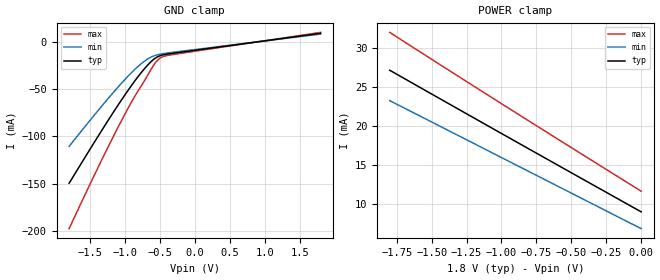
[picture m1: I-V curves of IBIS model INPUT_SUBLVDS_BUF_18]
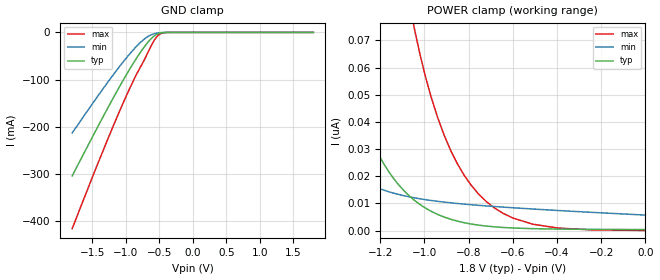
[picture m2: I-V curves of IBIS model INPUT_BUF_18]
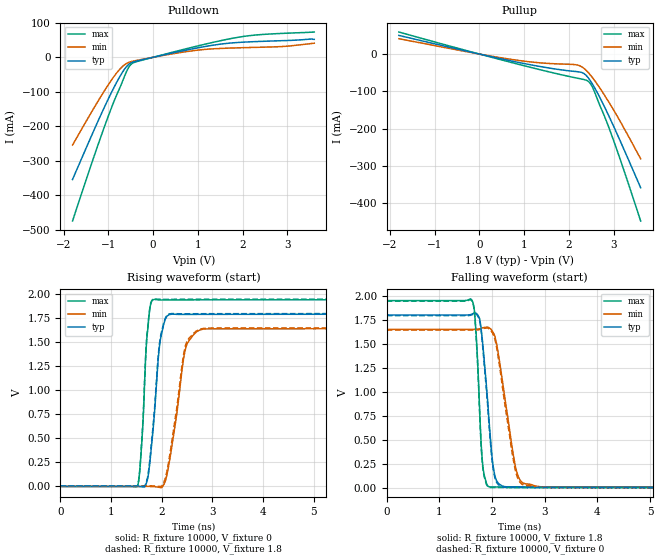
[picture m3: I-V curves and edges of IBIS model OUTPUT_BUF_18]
| TEXAS INSTRUMENTS INCORPORATED
| DLP Products
| IBIS Model of D4885XT7SV
| DLP2010 DMD
| This device can be powered at the following Vccs:
|  1.8 volt Vcc
| This file provides unique models under the [Model Selector] for each Vcc.
| For operation at a specific Vcc, select the appropriate model after each
| [Model Selector] keyword.
[IBIS Ver]   3.2
[Comment char]  |_char
[File Name]   dlp2010dmd_ibis.ibs
[File Rev]   1.0 | f_die
[Date]   December 3, 2012
[Source]   Data created from TI-SPICE simulations at TI-DLP.
[Notes]   The following is an IBIS list for the P2_WVGA.
##notes##|
[Disclaimer] Property of Texas Instruments Incorporated.  Unauthorized
   reproduction and/or distribution is strictly prohibited.
   This product is protected under copyright law.
   Created  2012, (C) Copyright  2012, Texas Instruments
   Incorporated, All Rights Reserved
   UNLESS THERE IS A SIGNED, WRITTEN AGREEMENT TO THE
   CONTRARY, TEXAS INSTRUMENTS (TI) IS PROVIDING THE IBIS
   MODELS  AND WITHOUT ANY WARRANTY, EXPRESSED OR
   IMPLIED.  TI assumes no liability for:
   1) the accuracy of the IBIS models provided to your
   company;
   2) the proper functioning of these IBIS Models in your
   design or for any resulting applications; or
   3) infringement of patents, copyrights or intellectual
   property rights resulting from your use of these IBIS
   models.
   TI provides IBIS Models as a service to our customers.
   You and your company shall not distribute, sell or give
   these models to anyone else without prior written
   permission from TI.
   TI reserves the right to make changes to our products or
   to discontinue any semiconductor product or service
   without notice, and advises our customers to obtain the
   latest version of relevant information to verify, before
   placing orders, that the information being relied on is
   current.
   Please be aware that your receipt and use of the IBIS
   information provided shall serve as acceptance of these
   terms and conditions.  If you do not accept these terms,
   you should return or destroy the IBIS models and any
   other accompanying information immediately.
| Component DLP2010 40-pin PGA
[Component]   DLP2010
[Manufacturer]   Texas Instruments, Inc.
[Package]
|   typ   min   max
R_pkg   1.276e+00   6.417e-01   1.439e+00
L_pkg   5.442e-09   3.319e-09   6.457e-09
C_pkg   2.002e-12   1.417e-12   2.333e-12
[Pin]   signal_name   model_name   R_pin   L_pin   C_pin
G1   VDDI   POWER
G2   VDDI   POWER
G3   D_P<0>   INPUT_SUB_LVDS_BUF   1.398e+00   5.548e-09   2.270e-12
G4   D_N<0>   INPUT_SUB_LVDS_BUF   1.425e+00   5.892e-09   2.333e-12
G5   VDDI   POWER
G6   VDDI   POWER
G7   D_P<1>   INPUT_SUB_LVDS_BUF   1.427e+00   6.052e-09   1.970e-12
G8   D_N<1>   INPUT_SUB_LVDS_BUF   1.439e+00   6.208e-09   1.878e-12
G9   VSS   GND
G10   VSS   GND
G11   LS_RDATA   OUTPUT_BUF   1.414e+00   6.457e-09   2.308e-12
G12   DMD_DEN_ARSTZ INPUT_BUF   9.967e-01   4.805e-09   1.900e-12
G13   VSS   GND
G14   VSS   GND
G15   VSS   GND
G16   VSS   GND
G17   VSS   GND
G18   LS_WDATA   INPUT_BUF   6.417e-01   3.319e-09   1.454e-12
G19   LS_CLK   INPUT_BUF   6.511e-01   3.395e-09   1.417e-12
G20   VDD   POWER
H1   D_N<3>   INPUT_SUB_LVDS_BUF   1.386e+00   5.227e-09   2.120e-12
H2   D_P<3>   INPUT_SUB_LVDS_BUF   1.404e+00   5.656e-09   1.942e-12
H3   VSS   GND
H4   VSS   GND
H5   D_N<2>   INPUT_SUB_LVDS_BUF   1.422e+00   5.823e-09   2.144e-12
H6   D_P<2>   INPUT_SUB_LVDS_BUF   1.413e+00   5.770e-09   2.030e-12
H7   VSS   GND
H8   VSS   GND
H9   DCLK_N   INPUT_SUB_LVDS_BUF   1.425e+00   5.952e-09   2.136e-12
H10   DCLK_P   INPUT_SUB_LVDS_BUF   1.428e+00   6.083e-09   2.128e-12
H11   VSS   GND
H12   VSS   GND
H13   VOFFSET   POWER
H14   VDD   POWER
H15   VDD   POWER
H16   VDD   POWER
H17   VBIAS   POWER
H18   VRESET   POWER
H19   VDD   POWER
H20   VDD   POWER
| NOTE:  The [Diff Pin] section is commented out because the ibischk3 program
|   currently flags it as an Error when it shouldn't
| [Diff Pin]  inv_pin   vdiff   tdelay_typ
|G3   G4   200mv   NA
|G7   G8   200mv   NA
|H6   H5   200mv   NA
|H2   H1   200mv   NA
|H10   H9   200mv   NA
| Model INPUT_SUB_LVDS_BUF
[Model Selector]   INPUT_SUB_LVDS_BUF
INPUT_SUBLVDS_BUF_18   1.8 volt Vcc
| Model INPUT_BUF
[Model Selector]   INPUT_BUF
INPUT_BUF_18   1.8 volt Vcc
| Model OUTPUT_BUF
[Model Selector]   OUTPUT_BUF
OUTPUT_BUF_18   1.8 volt Vcc
| Models and submodels in the file (3): INPUT_SUBLVDS_BUF_18 (Input), INPUT_BUF_18 (Input), OUTPUT_BUF_18 (Output)
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[Model]   INPUT_SUBLVDS_BUF_18
Model_type  Input
Vinl=0.80
Vinh=1.00
| variable   typ   min   max
C_comp   0.69pF   0.66pF   0.72pF
[Temperature Range]   25   85   -40
[Voltage range]   1.8   1.65   1.95
[GND Clamp]
| INPUT_SUBLVDS_BUF_18
|   Voltage   I(typ)   I(min)   I(max)
-1.8V     -149.7mA   -110.7mA   -197.8mA
-1.29V    -88.84mA   -64.29mA   -118.6mA
-1.095V   -66.55mA   -47.56mA   -89.83mA
-930mV    -48.67mA   -34.42mA   -66.87mA
-790mV    -34.7mA    -24.56mA   -49.3mA
-680mV    -25.03mA   -18.39mA   -35.98mA
-580mV    -18.08mA   -14.73mA   -23.73mA
-510mV    -15.09mA   -13.26mA   -17.94mA
-450mV    -13.75mA   -12.43mA   -15.53mA
-355mV    -12.57mA   -11.45mA   -13.96mA
1.8V      8.993mA    8.203mA    9.976mA
[POWER Clamp]
| INPUT_SUBLVDS_BUF_18
|   Voltage   I(typ)   I(min)   I(max)
-1.8V     27.16mA    23.26mA    32.02mA
-1.37V    22.79mA    19.34mA    27.08mA
-920mV    18.24mA    15.23mA    21.97mA
-16.28fV  8.993mA    6.835mA    11.65mA
[Model]   INPUT_BUF_18
Model_type  Input
Vinl=0.54
Vinh=1.26
| variable   typ   min   max
C_comp   0.51pF   0.44pF   0.58pF
[Temperature Range]   25   85   -40
[Voltage range]   1.8   1.65   1.95
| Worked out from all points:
|   GND clamp passes 1 mA (typ) near -0.47 V on its own axis
[GND Clamp]
| INPUT_BUF_18
|   Voltage   I(typ)   I(min)   I(max)
-1.8V     -304mA     -213.1mA   -415.8mA
-1.52V    -227.4mA   -155.6mA   -314.4mA
-1.29V    -165.7mA   -109.6mA   -233.4mA
-1.095V   -115.3mA   -72.59mA   -167.6mA
-930mV    -75.06mA   -43.75mA   -115.2mA
-790mV    -43.93mA   -22.51mA   -75.55mA
-680mV    -22.72mA   -9.755mA   -45.56mA
-580mV    -7.998mA   -2.996mA   -17.96mA
-510mV    -2.379mA   -972.8uA   -5.564mA
-450mV    -592.5uA   -304.6uA   -1.296mA
-355mV    -35.15uA   -32.8uA    -61.22uA
1.8V      384pA      6.33nA     42.47pA
[POWER Clamp]
| INPUT_BUF_18
|   Voltage   I(typ)   I(min)   I(max)
-1.8V     438.6nA    109.4nA    1.836uA
-1.7V     293.4nA    73.99nA    1.296uA
-1.565V   164.4nA    44.27nA    784.1nA
-1.4V     75.97nA    25.31nA    401.7nA
-1.255V   36.21nA    17.25nA    210.8nA
-1.155V   20.97nA    14.17nA    130.5nA
-1.045V   11.14nA    12.07nA    74.21nA
-970mV    7.14nA     11.1nA     49.29nA
-880mV    4.163nA    10.23nA    29.33nA
-685mV    1.408nA    8.888nA    8.453nA
-395mV    567.5pA    7.406nA    949.3pA
-16.28fV  384pA      5.724nA    60.79pA
[Model]   OUTPUT_BUF_18
Model_type  Output
Vref =   0
Rref =   10000
Cref =   10p
Vmeas =   1.2
| variable   typ   min   max
C_comp   0.65pF   0.45pF   1.15pF
| C_pullup   0.66pF   0.45pF   1.15pF
| C_pulldown   0.63pF   0.50pF   1.03pF
[Temperature Range]   25   85   -40
[Voltage range]   1.8   1.65   1.95
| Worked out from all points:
|   slope of the pulldown table from 0 to 0.27 V, typ, clamps not added: 34.3 ohm
|   slope of the pullup table from 0 to 0.27 V, typ, clamps not added: 37.6 ohm
|   rising waveform, R_fixture 10000, V_fixture 0: 20-80 % time 164ps typ, 253ps min, 111ps max; typ from 0 V to 1.79 V
|   falling waveform, R_fixture 10000, V_fixture 1.8: 20-80 % time 159ps typ, 266ps min, 98.4ps max; typ from 1.8 V to 0.006 V
|   rising waveform, R_fixture 10000, V_fixture 1.8: 20-80 % time 164ps typ, 256ps min, 110ps max; typ from 0.006 V to 1.8 V
|   falling waveform, R_fixture 10000, V_fixture 0: 20-80 % time 159ps typ, 263ps min, 98.5ps max; typ from 1.79 V to 0 V
[Pulldown]
| OUTPUT_BUF_18
|   Voltage   I(typ)   I(min)   I(max)
-1.8V     -354.2mA   -254.4mA   -474.4mA
-1.265V   -195mA     -134.5mA   -266.6mA
-895mV    -92.67mA   -59.47mA   -134.6mA
-755mV    -58.61mA   -36.11mA   -91.94mA
-645mV    -35.65mA   -22.4mA    -56.96mA
-555mV    -21.67mA   -15.53mA   -31.37mA
-480mV    -15.3mA    -12.24mA   -19.11mA
-345mV    -10.18mA   -8.457mA   -11.8mA
875mV     24.33mA    18.74mA    29.04mA
1.865V    42.67mA    27.28mA    57.21mA
2.905V    48.22mA    31.33mA    69.32mA
3.6V      52.02mA    40.86mA    73.18mA
[Pullup]
| OUTPUT_BUF_18
|   Voltage   I(typ)   I(min)   I(max)
-1.8V     49.99mA    41.08mA    59.07mA
730mV     -18.9mA    -14.55mA   -23.06mA
1.36V     -33.47mA   -23.55mA   -42.08mA
2.165V    -46.93mA   -28.87mA   -64.13mA
2.32V     -51.32mA   -37.02mA   -67.96mA
2.435V    -64.68mA   -50.22mA   -73.6mA
2.49V     -74.19mA   -58.09mA   -81.45mA
2.545V    -84.87mA   -66.63mA   -94.28mA
2.7V      -119.1mA   -93.19mA   -140.9mA
2.895V    -167.2mA   -129.8mA   -198.5mA
3.195V    -246.7mA   -191.5mA   -300.4mA
3.6V      -358.2mA   -280.8mA   -447.3mA
[Ramp]
| OUTPUT_BUF_18
| variable   typ   min   max
dV/dt_r   1.08/1.67E-10   0.99/2.58E-10   1.17/1.11E-10
dV/dt_f   1.09/1.62E-10   1.00/2.72E-10   1.18/1.01E-10
R_load = 10000
[Rising Waveform]
| OUTPUT_BUF_18
R_fixture =   10000
C_fixture =   0
L_fixture =   0
V_fixture =   0
V_fixture_min = 0
V_fixture_max = 0
|   Time   V(typ)   V(min)   V(max)
0s        2.935nV    32.33nV    304.2pV
1.525ns   12.81uV    20.21uV    4.084mV
1.615ns   -3.833mV   105uV      533.5mV
1.71ns    58.13mV    123.1uV    1.568V
1.855ns   750.8mV    -2.782mV   1.947V
1.955ns   1.458V     -9.919mV   1.942V
2.08ns    1.753V     73.73mV    1.941V
2.47ns    1.791V     1.436V     1.942V
2.825ns   1.792V     1.638V     1.943V
24.99ns   1.793V     1.642V     1.944V
[Falling Waveform]
| OUTPUT_BUF_18
R_fixture =   10000
C_fixture =   0
L_fixture =   0
V_fixture =   1.8
V_fixture_min = 1.65
V_fixture_max = 1.95
|   Time   V(typ)   V(min)   V(max)
0s        1.8V       1.65V      1.95V
1.62ns    1.81V      1.65V      1.949V
1.69ns    1.819V     1.651V     1.653V
1.76ns    1.764V     1.656V     844.3mV
1.82ns    1.507V     1.667V     244.5mV
1.955ns   601.1mV    1.662V     9.6mV
2.08ns    79.45mV    1.512V     9.328mV
2.475ns   9.39mV     152mV      8.293mV
2.885ns   8.404mV    13.17mV    7.567mV
24.99ns   6.04mV     6.675mV    5.66mV
[Rising Waveform]
| OUTPUT_BUF_18
R_fixture =   10000
C_fixture =   0
L_fixture =   0
V_fixture =   1.8
V_fixture_min = 1.65
V_fixture_max = 1.95
|   Time   V(typ)   V(min)   V(max)
0s        6.039mV    6.675mV    5.66mV
1.525ns   6.058mV    6.695mV    10.55mV
1.61ns    2.738mV    6.771mV    514.5mV
1.71ns    72.65mV    6.795mV    1.588V
1.855ns   789.8mV    4.171mV    1.952V
1.955ns   1.486V     187.2uV    1.948V
2.08ns    1.761V     104.7mV    1.948V
2.465ns   1.798V     1.459V     1.948V
2.825ns   1.798V     1.646V     1.949V
24.99ns   1.8V       1.65V      1.95V
[Falling Waveform]
| OUTPUT_BUF_18
R_fixture =   10000
C_fixture =   0
L_fixture =   0
V_fixture =   0
V_fixture_min = 0
V_fixture_max = 0
|   Time   V(typ)   V(min)   V(max)
0s        1.793V     1.642V     1.944V
1.62ns    1.803V     1.642V     1.942V
1.69ns    1.811V     1.643V     1.63V
1.76ns    1.748V     1.648V     814.7mV
1.815ns   1.504V     1.657V     253.2mV
1.955ns   560.3mV    1.649V     4.112mV
2.075ns   66.14mV    1.49V      3.651mV
2.465ns   3.348mV    135.5mV    2.653mV
2.86ns    2.404mV    7.718mV    1.943mV
24.99ns   6.498nV    37.43nV    3.212nV
